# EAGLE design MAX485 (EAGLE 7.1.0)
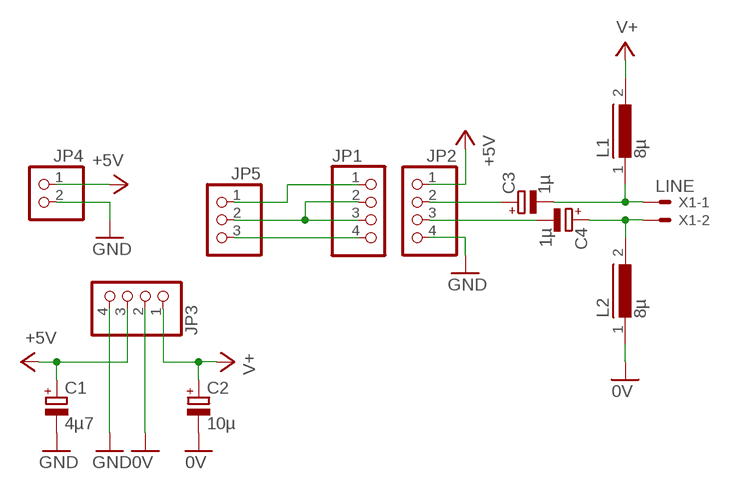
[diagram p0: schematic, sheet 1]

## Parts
C1  4µ7  CPOL-EUE2.5-6  [E2,5-6]
C2  10µ  CPOL-EUE2.5-6  [E2,5-6]
C3  1µ  CPOL-EUE2-5  [E2-5]
C4  1µ  CPOL-EUE2-5  [E2-5]
JP1  PINHD-1X4  [1X04]
JP2  PINHD-1X4  [1X04]
JP3  PINHD-1X4  [1X04]
JP4  PINHD-1X2  [1X02]
JP5  PINHD-1X3  [1X03]
L1  8µ  82114A  [82114A]
L2  8µ  82114A  [82114A]
X1  LINE  22-23-2021  [22-23-2021]

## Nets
0V: C2.- JP3.2 L2.1
+5V: C1.+ JP2.1 JP3.3 JP4.1
GND: C1.- JP2.4 JP3.4 JP4.2
N$1: C4.+ L2.2 X1.2
N$2: C3.- L1.1 X1.1
N$3: JP1.2 JP1.3 JP5.2
N$4: JP1.4 JP5.3
N$5: JP1.1 JP5.1
N$9: C3.+ JP2.2
N$10: C4.- JP2.3
V+: C2.+ JP3.1 L1.2

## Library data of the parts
C1-C4 = rcl:CPOL-EU: POLARIZED CAPACITOR, European symbol
JP1-JP3 = pinhead:PINHD-1X4: PIN HEADER
JP4 = pinhead:PINHD-1X2: PIN HEADER
JP5 = pinhead:PINHD-1X3: PIN HEADER
L1 L2 = inductors:82114A: INDUCTOR
X1 = con-molex:22-23-2021: .100" (2.54mm) Center Header - 2 Pin; MF: MOLEX; MPN: 22-23-2021; OC_FARNELL: 1462926; OC_NEWARK: 25C3832

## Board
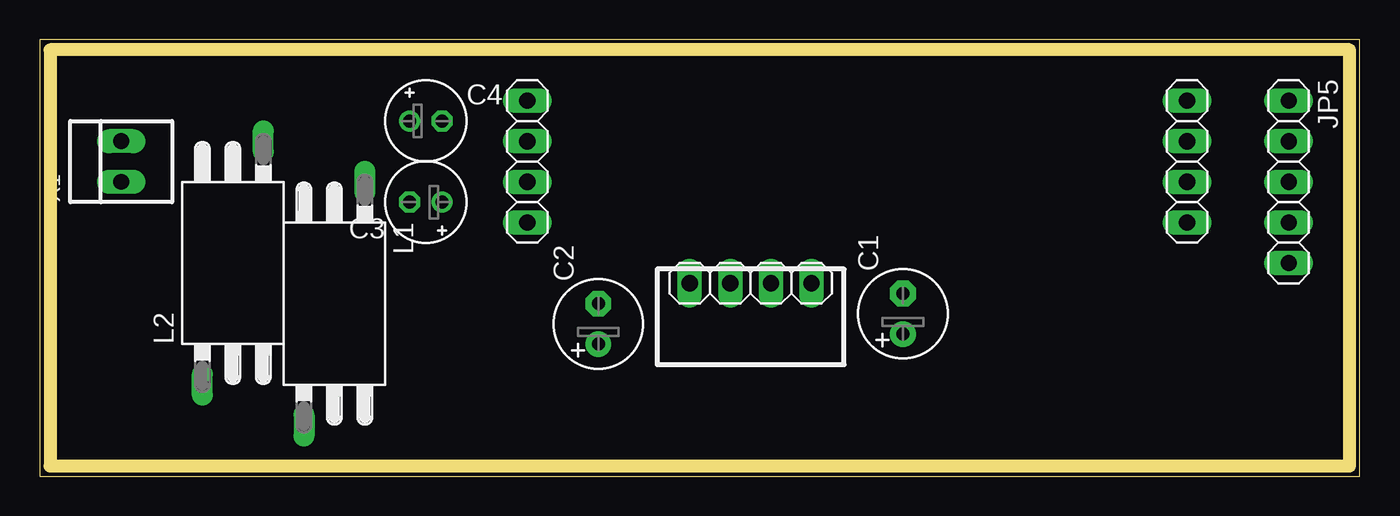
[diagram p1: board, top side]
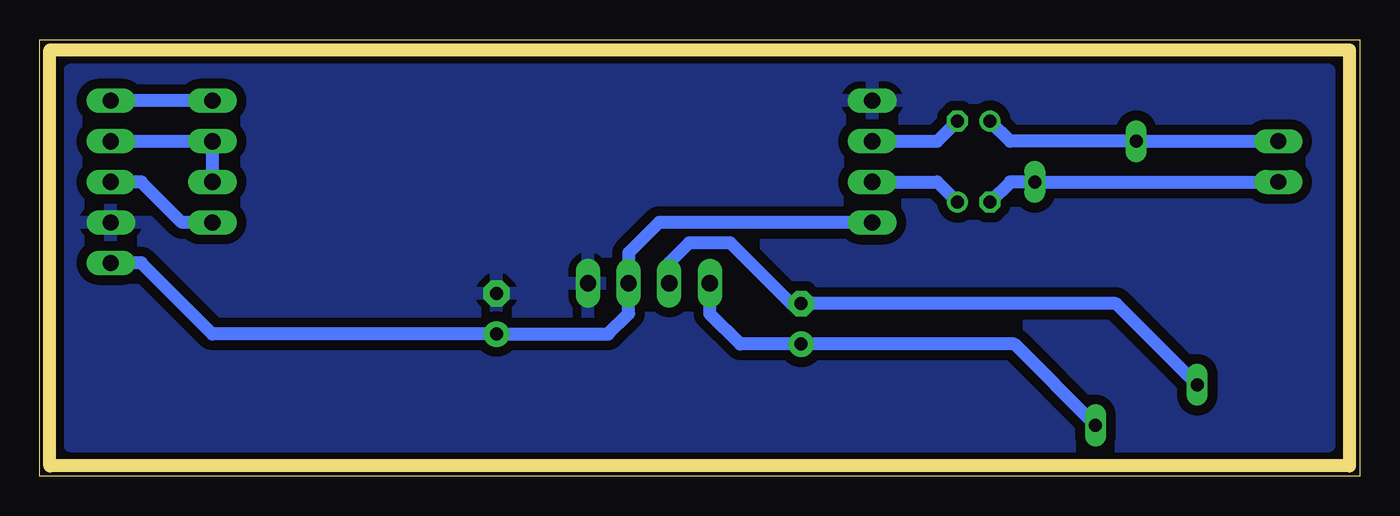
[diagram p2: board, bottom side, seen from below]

Size 82.54 x 27.3 mm. Coordinates in mm from the lower left corner, seen from the top.
Outline: 0,0 82.54,0 82.54,27.3 0,27.3 0,0
Copper layers (1*16): Top 0.035mm / dielectric 1.5mm / Bottom 0.035mm
Design rules "default *": minimum track width 10mil, minimum drill 24mil, track to track 8mil, track to pad 8mil, pad to pad 8mil, via to via 8mil, smd to smd 8mil, copper to edge 40mil, drill to drill 8mil, minimum pad ring 10mil, minimum via ring 8mil, stop-mask expansion 4mil, vias tented up to drill 0mil, thermal gap 18mil
Milling: 4 lines

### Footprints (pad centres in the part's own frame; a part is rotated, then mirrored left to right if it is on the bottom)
E2,5-6 = drill 0.813 pad 1.6: + -1.27,0 | drill 0.813 pad 1.6 octagon: - 1.27,0
E2-5 = drill 0.813 pad 1.27: + -1.016,0 | drill 0.813 pad 1.27 octagon: - 1.016,0
1X04 = drill 1.016 long: 1 -3.81,0; 2 -1.27,0; 3 1.27,0; 4 3.81,0
1X02 = drill 1.016 long: 1 -1.27,0; 2 1.27,0
1X03 = drill 1.016 long: 1 -2.54,0; 2 0,0; 3 2.54,0
82114A = drill 0.813 long: 1 -7.62,1.905; 2 7.62,-1.905
22-23-2021 = drill 1 long: 1 -1.27,0; 2 1.27,0

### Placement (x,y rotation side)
C1  53.98,10.16 90 top
C2  34.92,9.53 90 top
C3  24.13,17.14 180 top
C4  24.13,22.23 0 top
JP1  71.75,19.68 270 top
JP2  30.48,19.68 90 top
JP3  44.45,12.06 0 top
JP4  78.11,14.61 90 top
JP5  78.11,20.95 270 top
L1  18.41,10.79 270 top
L2  12.06,13.34 90 top
X1  5.08,19.68 90 top

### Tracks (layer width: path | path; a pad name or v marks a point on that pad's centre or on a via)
0V
  Bottom 0.813: L2.1 15.24,10.79 C2.- 35.56,10.79 39.37,14.61 41.91,14.61 43.18,13.34 JP3.2
+5V
  Bottom 0.813: JP2.1 43.81,15.88 45.72,13.97 JP3.3 45.72,10.16 46.99,8.89 C1.+ 71.75,8.89 76.2,13.34 JP4.1
GND
  pour Bottom (isolate 0.61): 1.91,25.4 80.64,25.4 80.64,1.91 1.91,1.91
N$1
  Bottom 0.813: C4.+ 21.84,20.95 L2.2 X1.2
N$2
  Bottom 0.813: C3.- 21.84,18.41 L1.1 X1.1
N$3
  Bottom 0.813: JP1.3 JP1.2 JP5.2
N$4
  Bottom 0.813: JP1.4 73.66,15.88 76.2,18.41 JP5.3
N$5
  Bottom 0.813: JP1.1 JP5.1
N$9
  Bottom 0.813: JP2.2 26.42,18.41 C3.+
N$10
  Bottom 0.813: JP2.3 26.42,20.95 C4.-
V+
  Bottom 0.813: JP3.1 40.64,10.16 38.73,8.26 C2.+ 21.59,8.26 L1.2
